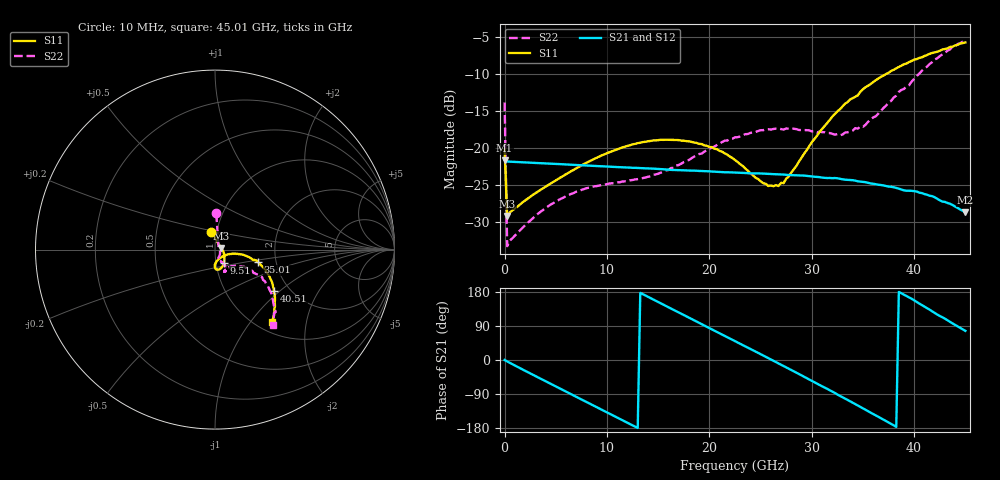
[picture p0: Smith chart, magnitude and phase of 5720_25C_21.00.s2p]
! Device:  ADRF5720
! Description: 0.5dB LSB GaAs MMIC 6-bit Digital Attenuator
! Frequency:  0.000009 -  40 GHz
! Ports:
!	RF1	= Port 1
!	RF2	= Port 2
! Vdd:  3.3 Volt
! Vss:  -3.3 Volt
! Control:  0/3.3 Volt
! State:  21.00 dB attenuation
! Data:  The device was measured using G-S-G Probes on a matrix board.
!  Data was collected using an calibrated 4 port network analyzer.
!  The reference plane for this measurement is at the launchers.
! Note:  Analog Devices supplies this data as a sample of measured data
!  for this product.  Your particular data for this product may vary.
!  Data was taken at 25 degrees C.
!  Analog Devices reserves the right to change this data at anytime.
# GHZ S DB R 45.0
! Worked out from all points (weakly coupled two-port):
!   181 points, 10 MHz to 45.01 GHz, reference 45 ohm
!   highest |S21| = -21.66 dB at 10 MHz (marker M1); lowest = -28.7 dB at 45.01 GHz (marker M2)
!   lowest |S11| = -29.2 dB at 260 MHz (marker M3), VSWR 1.07, Z = 48.1 + j0.87 ohm
!   |S11| at or under -10 dB: start of sweep to 37.33 GHz
!   |S22| runs from -33.3 to -5.5 dB; largest |S21 - S12| = 0.00012
!   S11 on the Smith chart (normalised r, x): 10 MHz: 0.94, +0.18; 9.51 GHz: 1.09, -0.16; 35.01 GHz: 1.61, -0.23; 40.51 GHz: 1.67, -0.92; 45.01 GHz: 1.16, -1.28
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0.01  -20.20 102.0  -21.66 0.0  -21.66 0.1  -13.89 88.0
0.26  -29.20 15.1  -21.85 -3.9  -21.85 -3.9  -33.27 21.8
1.26  -27.95 0.1  -21.92 -18.0  -21.92 -18.0  -31.47 -8.3
3.51  -25.68 -19.7  -22.07 -49.2  -22.07 -49.2  -28.64 -41.7
5.01  -24.39 -31.0  -22.17 -69.8  -22.17 -69.8  -27.23 -56.1
7.76  -22.19 -47.1  -22.37 -107.5  -22.37 -107.5  -25.56 -70.8
9.51  -21.01 -55.8  -22.49 -131.4  -22.49 -131.4  -25.02 -74.9
12.51  -19.54 -68.5  -22.70 -172.5  -22.70 -172.5  -24.34 -74.0
15.26  -18.92 -78.2  -22.86 149.4  -22.86 149.4  -23.35 -66.9
19.26  -19.49 -88.7  -23.13 94.5  -23.13 94.5  -20.78 -58.9
21.26  -20.53 -90.6  -23.27 66.9  -23.27 66.9  -19.21 -59.1
22.76  -21.92 -89.7  -23.36 46.3  -23.36 46.3  -18.57 -60.2
25.26  -24.77 -70.1  -23.48 11.8  -23.48 11.8  -17.62 -63.9
26.76  -25.15 -45.9  -23.58 -9.0  -23.58 -8.9  -17.38 -65.0
27.76  -23.88 -29.3  -23.67 -23.0  -23.67 -23.0  -17.42 -66.2
30.26  -18.82 -11.2  -23.90 -58.5  -23.89 -58.5  -17.78 -65.1
32.76  -14.79 -11.8  -24.18 -94.7  -24.19 -94.6  -18.31 -55.9
35.01  -12.09 -16.0  -24.61 -127.5  -24.61 -127.5  -17.17 -41.0
37.76  -9.64 -25.4  -25.26 -168.5  -25.26 -168.4  -13.67 -29.5
40.51  -7.88 -35.1  -26.05 148.9  -26.05 148.9  -10.00 -32.2
43.76  -6.35 -46.9  -27.72 96.5  -27.72 96.4  -6.29 -45.7
45.01  -5.79 -52.1  -28.71 76.8  -28.70 76.9  -5.52 -52.4
